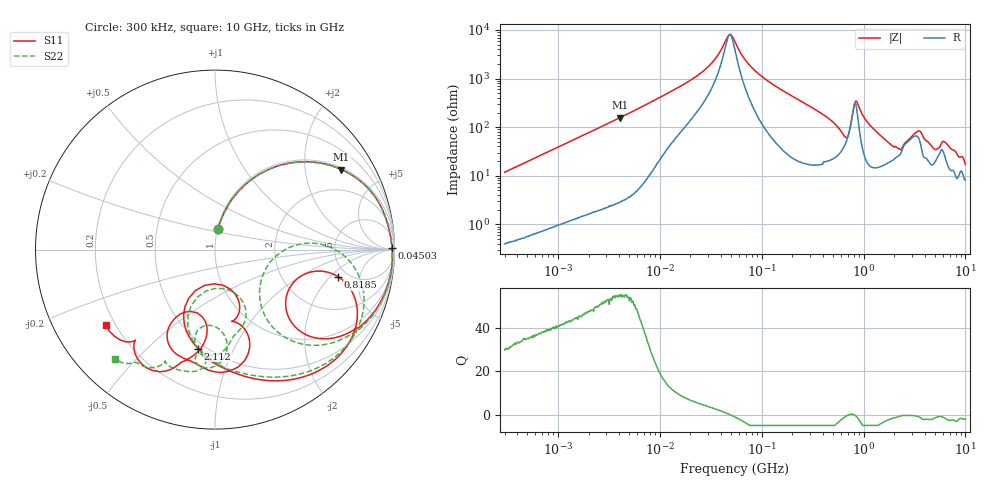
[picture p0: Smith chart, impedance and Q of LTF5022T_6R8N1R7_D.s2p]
! S-Parameter Data Generated by TDK Corporation
! Copyright(C) 2020 TDK Corporation.
! All Rights Reserved.
! TDK P/N: LTF5022T-6R8N1R7-D (Inductor)
! Property: L=6.8uH at 100kHz
! Size(LxWxT): 6.5x5x2.2mm
! Model Type: s2p (Touchstone File Format Version 1.0)
! Frequency: DC=Yes Start=0.3MHz Stop=10000MHz 802points Log-sweep
! Model Generated on Apr. 23, 2020
! Port Assignments:
!  1 ---@@@--- 2
! Applicable Conditions:
!  Temperature = 25 degC
!  DC Bias Current = 0 A
!  Small Signal Operation
! Terms and conditions regarding TDK Simulation Models
! (1)This simulation model is being provided solely for informational purposes. Please refer to the specifications of the products in terms of detailed characteristics of such products.
! (2)In no event shall TDK Corporation of any of its subsidiaries be liable for any loss or damage arising, directly or indirectly,
!  From any information contained in this simulation model, including, but not limited to loss or damages arising from any inaccuracies, omissions or errors in connection with such information.
! (3)Any and all copyrights on this simulation model are owned by TDK Corporation.
!  Duplication or redistribution of this simulation model without prior written permission from TDK Corporation is prohibited.
! (4)This simulation model is subject to any modification or change without any prior notice.
! (5)Neither TDK Corporation nor any of its subsidiaries shall make any warranty, express or implied,
!  Including but not limited to the correctness, implied warranties of merchantability and fitness for a particular purpose with respect to this simulation models.
! (6)The use of this simulation model shall be deemed to have consented to the terms and conditions hereof.
# Hz S MA R 50
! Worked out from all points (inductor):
!   801 points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, 300 kHz to 10 GHz, reference 50 ohm
!   read as 1/Y11, port 2 shorted: L = 6.24 uH near 318.3 kHz
!   highest Q = 54.7 at 4.054 MHz (marker M1), where L = 6.13 uH
!   self-resonance near 48.75 MHz
!   S11 on the Smith chart (normalised r, x): 300 kHz: 1.01, +0.24; 45.03 MHz: open; 818.5 MHz: 4.18, -2.49; 2.112 GHz: 0.46, -0.74; 10 GHz: 0.16, -0.30
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300000  0.117 81.4  0.9893 -6.7  0.9891 -6.7  0.1169 81.3
1713600  0.5443 55.7  0.8269 -33.0  0.8269 -33.0  0.5441 55.7
4053600  0.8341 32.3  0.5365 -56.6  0.5366 -56.6  0.8341 32.3
9671944  0.957 14.1  0.2479 -73.2  0.2479 -73.2  0.9571 14.0
4.503434e7  0.9869 0.5  0.03308 -67.4  0.03307 -67.4  0.9869 0.3
5.477226e7  0.9882 -0.8  0.01812 -51.2  0.01812 -51.1  0.9883 -0.9
6.736104e7  0.9892 -2.1  0.01126 16.4  0.01125 16.4  0.9892 -2.4
1.063884e8  0.9895 -5.6  0.04693 72.7  0.04692 72.7  0.9895 -6.0
3.126428e8  0.9504 -21.7  0.2276 61.4  0.2276 61.4  0.9483 -23.3
5.285151e8  0.7822 -39.4  0.454 32.2  0.454 32.2  0.7593 -44.6
6.738867e8  0.4998 -38.0  0.6073 -4.8  0.6074 -4.8  0.3751 -48.1
8.18524e8  0.7028 -12.4  0.4216 -54.9  0.4216 -55.0  0.6201 2.1
1.024756e9  0.9108 -36.0  0.07863 -27.0  0.07848 -26.8  0.905 -26.7
1.767019e9  0.6747 -84.0  0.3801 -17.8  0.3818 -17.9  0.7221 -74.8
2.112126e9  0.5597 -99.6  0.3495 -41.4  0.3528 -41.9  0.6007 -93.8
2.477118e9  0.2055 -76.5  0.3686 -10.4  0.3586 -10.5  0.2297 -73.4
3.219363e9  0.412 -76.2  0.4788 -77.2  0.4757 -76.9  0.5041 -79.1
3.991169e9  0.6803 -90.6  0.3103 -89.8  0.3107 -90.0  0.4666 -102.5
4.982529e9  0.572 -117.5  0.2317 -124.9  0.2355 -123.8  0.6394 -88.4
7.06055e9  0.6232 -103.4  0.3014 -176.3  0.2986 -176.0  0.6998 -109.9
8.993752e9  0.676 -131.3  0.1347 102.4  0.1372 103.6  0.7647 -124.0
1e10  0.74 -145.4  0.01985 -51.6  0.01737 -57.2  0.824 -132.5
